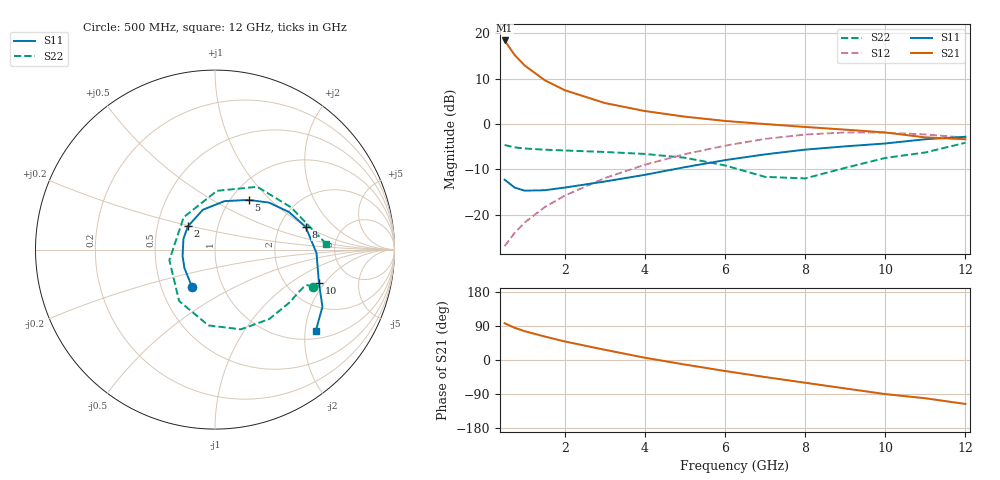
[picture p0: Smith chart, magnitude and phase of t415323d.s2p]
!AT-41532
!S-PARAMETERS at Vce=2.7V  Ic=10mA.  LAST UPDATED 05-29-98
# ghz s ma r 50
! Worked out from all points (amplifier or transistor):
!   15 points, 500 MHz to 12 GHz, reference 50 ohm
!   highest |S21| = 18.4 dB at 500 MHz (marker M1)
!   |S21| within 3 dB of that: start of sweep to 734.6 MHz
!   unconditionally stable (mu >= 1): 710.4 MHz to 2.262 GHz
!   at 1 GHz: K = 1.04, MAG = 16.0 dB, |S12| = -21.7 dB
!   at 5 GHz: K = 0.84, MSG = 4.1 dB, |S12| = -6.7 dB
!   at 12 GHz: K = 0.99, MSG = -0.2 dB, |S12| = -3.0 dB
!   S11 on the Smith chart (normalised r, x): 500 MHz: 0.71, -0.31; 2 GHz: 0.72, +0.19; 5 GHz: 1.20, +0.75; 8 GHz: 2.80, +0.97; 10 GHz: 2.96, -1.77; 12 GHz: 1.20, -2.28
0.5  0.243 -122.0  8.31 97.0  0.045 68.0  0.586 -21.0
0.75  0.199 -149.0  5.751 85.0  0.063 69.0  0.552 -21.0
1  0.184 -169.0  4.408 76.0  0.082 69.0  0.536 -23.0
1.5  0.186 161.0  3.034 62.0  0.121 67.0  0.52 -28.0
2  0.199 139.0  2.354 49.0  0.162 63.0  0.51 -35.0
3  0.232 107.0  1.7 27.0  0.253 52.0  0.491 -52.0
4  0.275 79.0  1.387 6.0  0.355 39.0  0.467 -72.0
5  0.334 56.0  1.202 -12.0  0.465 24.0  0.424 -95.0
6  0.399 41.0  1.079 -29.0  0.576 7.0  0.349 -125.0
7  0.462 27.0  0.997 -45.0  0.684 -12.0  0.261 -167.0
8  0.521 14.0  0.926 -60.0  0.764 -32.0  0.251 134.0
9  0.566 -2.0  0.865 -75.0  0.805 -52.0  0.328 88.0
10  0.609 -18.0  0.805 -90.0  0.802 -72.0  0.422 56.0
11  0.678 -28.0  0.711 -101.0  0.766 -91.0  0.485 29.0
12  0.722 -39.0  0.678 -116.0  0.706 -106.0  0.62 3.0
